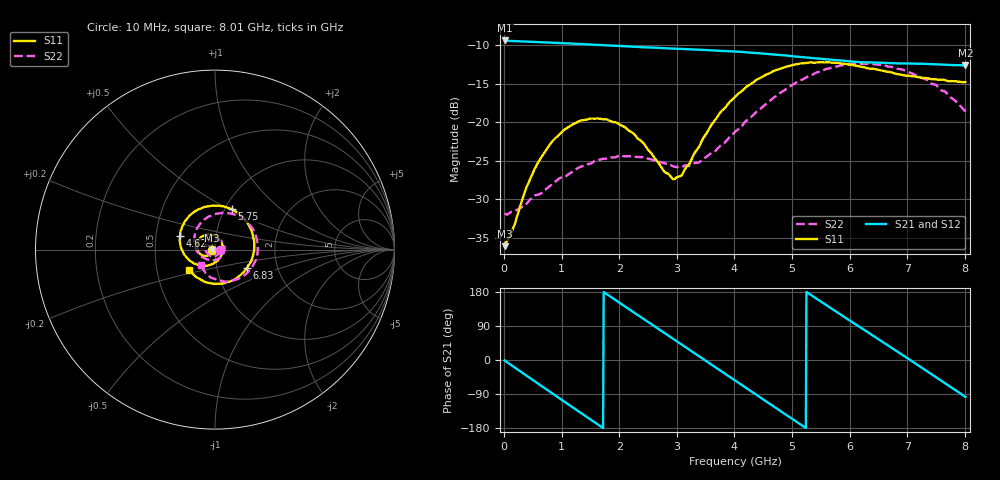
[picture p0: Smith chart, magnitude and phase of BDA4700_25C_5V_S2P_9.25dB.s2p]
!Agilent Technologies,E5071B,MY42404982,A.09.10
!Date: Mon Oct 20 13:30:39 2025
!Data & Calibration Information:
!Freq	S11:SOLT2(ON)	S21:SOLT2(ON)	S12:SOLT2(ON)	S22:SOLT2(ON)
# Hz S RI R 50
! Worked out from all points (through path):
!   801 points, 10 MHz to 8.01 GHz, reference 50 ohm
!   highest |S21| = -9.37 dB at 20 MHz (marker M1); lowest = -12.6 dB at 8.01 GHz (marker M2)
!   group delay of S21, straight-line fit = 283 ps
!   lowest |S11| = -36.1 dB at 10 MHz (marker M3), VSWR 1.03, Z = 48.5 - j0.135 ohm
!   |S11| at or under -10 dB: start of sweep to end of sweep
!   |S22| runs from -32.0 to -12.4 dB; largest |S21 - S12| = 0.0024
!   S11 on the Smith chart (normalised r, x): 10 MHz: 0.97, -0.00; 4.62 GHz: 0.67, +0.11; 5.75 GHz: 1.08, +0.52; 6.83 GHz: 1.40, -0.29; 8.01 GHz: 0.73, -0.17
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1e7  -0.0156 -0.00139  0.3398 -0.00734  0.3398 -0.00772  0.0256 -0.0014
2e7  -0.0162 -0.0022  0.3397 -0.0133  0.3396 -0.0144  0.0254 -0.00149
3.4e8  -0.0243 -0.0231  0.2703 -0.1974  0.2703 -0.1976  0.0213 -0.0191
7.2e8  -0.0548 -0.0354  0.0803 -0.3202  0.0803 -0.3203  -0.00104 -0.0366
1.03e9  -0.0858 -0.021  -0.1014 -0.3101  -0.1017 -0.31  -0.0291 -0.033
1.35e9  -0.102 0.0145  -0.2515 -0.2011  -0.2516 -0.2012  -0.0513 -0.00607
1.93e9  -0.0603 0.0797  -0.2928 0.1137  -0.2927 0.1138  -0.0251 0.0536
2.32e9  -0.00385 0.0785  -0.1486 0.2704  -0.1487 0.2705  0.0221 0.0554
2.68e9  0.0361 0.0409  0.0419 0.3015  0.0419 0.3014  0.0513 0.0207
2.93e9  0.0429 0.000396  0.1659 0.2514  0.1659 0.251  0.0508 -0.0103
3.07e9  0.0383 -0.0235  0.2219 0.2014  0.2209 0.2022  0.0434 -0.0276
3.53e9  -0.0229 -0.0834  0.2932 -0.0236  0.2934 -0.0241  -0.0096 -0.0596
4.01e9  -0.1283 -0.0698  0.1704 -0.2323  0.1706 -0.2321  -0.079 -0.035
4.62e9  -0.195 0.0758  -0.1227 -0.2481  -0.1225 -0.2483  -0.1133 0.079
5e9  -0.1468 0.1836  -0.2436 -0.1134  -0.2443 -0.1137  -0.0669 0.1611
5.35e9  -0.0459 0.24  -0.2571 0.048  -0.2573 0.0473  0.0231 0.2014
5.75e9  0.0941 0.2253  -0.1606 0.1961  -0.1603 0.1963  0.143 0.1794
6.19e9  0.1995 0.1138  0.0181 0.245  0.0202 0.2454  0.2302 0.0681
6.68e9  0.2053 -0.0546  0.1936 0.1459  0.1941 0.1456  0.2146 -0.0822
6.83e9  0.1792 -0.1006  0.2234 0.0906  0.2241 0.0898  0.1881 -0.1196
7.34e9  0.0391 -0.1895  0.2088 -0.1169  0.2088 -0.1171  0.0593 -0.1796
8.01e9  -0.1442 -0.1118  -0.0303 -0.2322  -0.0297 -0.2326  -0.0777 -0.0882
